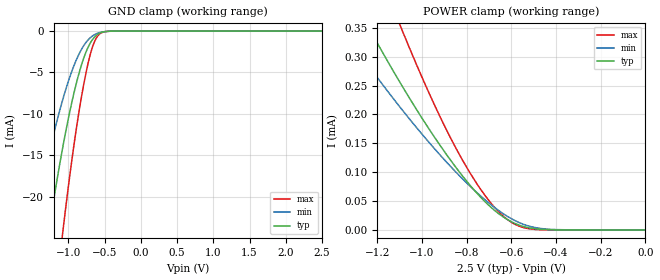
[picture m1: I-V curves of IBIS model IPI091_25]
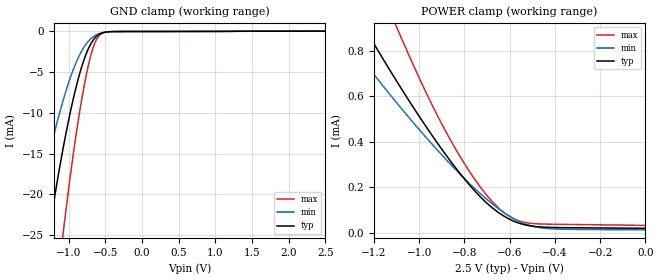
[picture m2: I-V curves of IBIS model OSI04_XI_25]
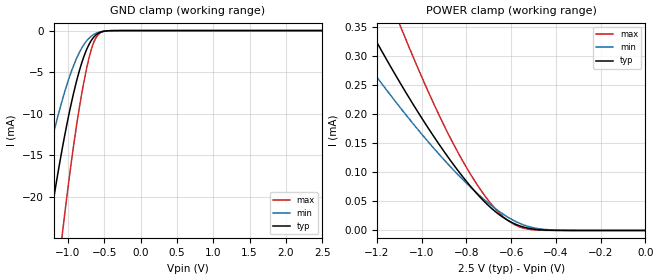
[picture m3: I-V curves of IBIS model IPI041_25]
| TEXAS INSTRUMENTS INCORPORATED
| Connectivity Solutions Group
| IBIS Model of TL16C752CRHB_2.5V
| 752C_RHB_2.5V
| This file contains package information for the following:
|  RHB 32-pin (QFN) package as [Component] 752CRHB_2.5V
| This device can be powered at the following Vccs:
|  2.5 Volt Vcc
| This file provides unique models under the [Model Selector] for each Vcc.
| For operation at a specific Vcc, select the appropriate model after each
| [Model Selector] keyword.
[IBIS Ver]   3.2
[Comment char]  |_char
[File Name]   752c_rhb_2_5v.ibs
[File Rev]   1 | a
[Date]   March 15, 2008
[Source]   Data created from TI-SPICE simulations at TI-CONN.
[Notes]   The following is an IBIS list for the 752C_RHB_2.5V.
   Please contact s-ly@ti.com with questions and
   comments concerning CONN IBIS models.
[Disclaimer] Property of Texas Instruments Incorporated.  Unauthorized
   reproduction and/or distribution is strictly prohibited.
   This product is protected under copyright law.
   Created  2003, (C) Copyright  2003, Texas Instruments
   Incorporated, All Rights Reserved
   UNLESS THERE IS A SIGNED, WRITTEN AGREEMENT TO THE
   CONTRARY, TEXAS INSTRUMENTS (TI) IS PROVIDING THE IBIS
   MODELS  AND WITHOUT ANY WARRANTY, EXPRESSED OR
   IMPLIED.  TI assumes no liability for:
   1) the accuracy of the IBIS models provided to your
   company;
   2) the proper functioning of these IBIS Models in your
   design or for any resulting applications; or
   3) infringement of patents, copyrights or intellectual
   property rights resulting from your use of these IBIS
   models.
   TI provides IBIS Models as a service to our customers.
   You and your company shall not distribute, sell or give
   these models to anyone else without prior written
   permission from TI.
   TI reserves the right to make changes to our products or
   to discontinue any semiconductor product or service
   without notice, and advises our customers to obtain the
   latest version of relevant information to verify, before
   placing orders, that the information being relied on is
   current.
   Please be aware that your receipt and use of the IBIS
   information provided shall serve as acceptance of these
   terms and conditions.  If you do not accept these terms,
   you should return or destroy the IBIS models and any
   other accompanying information immediately.
| Component 752C_2.5V_RHB 32-pin QFN
[Component]   752C_RHB_2.5V
[Manufacturer]   Texas Instruments, Inc.
[Package]
|   typ   min   max
R_pkg   0.03169   0.03002   0.03704
L_pkg   2.02289n   1.83543n   2.62435n
C_pkg   0.52087p   0.46196p   0.61212p
[Pin]   signal_name   model_name   R_pin   L_pin   C_pin
1   D6   IPI04_OPJ43   0.03132   1.96376n   0.50826p
2   D7   IPI04_OPJ43   0.03166   2.03022n   0.52764p
3   RXB   IPI041   0.03222   2.12197n   0.55702p
4   RXA   IPI041   0.03290   2.21862n   0.57989p
5   TXA   OPJ430   0.03010   1.83593n   0.46505p
6   TXB   OPJ430   0.03096   1.92107n   0.49718p
7   CSA   IPI041   0.03104   1.92183n   0.49798p
8   CSB   IPI041   0.03110   1.96691n   0.51031p
9   XTAL1   OSI04_XI   0.03077   1.83703n   0.47632p
10   XTAL2   OSI04   0.03175   1.92839n   0.50935p
11   IOW   IPI041   0.03007   1.83565n   0.46474p
12   GND   GND   0.03265   2.22076n   0.58208p
13   IOR   IPI041   0.03002   1.83657n   0.46196p
14   RTSB   OPJ430   0.03190   2.11324n   0.55339p
15   CTSB   IPI041   0.03704   2.62435n   0.54475p
16   A2   IPI041   0.03147   1.97163n   0.51867p
17   A1   IPI041   0.03142   1.92513n   0.50753p
18   A0   IPI041   0.03060   1.83543n   0.47574p
19   INTB   OPJ430   0.03159   2.04484n   0.53228p
20   INTA   OPJ430   0.03117   1.96768n   0.51149p
21   RTSA   OPJ430   0.03153   2.03432n   0.53110p
22   DTRA   OPJ430   0.03280   2.22331n   0.58366p
23   DTRB   OPJ430   0.03352   2.34940n   0.60960p
24   RESET   IPI091   0.03188   1.96764n   0.51741p
25   CTSA   IPI041   0.03373   2.35631n   0.61212p
26   VCC   POWER   0.03224   2.13122n   0.55769p
27   D0   IPI04_OPJ43   0.03191   2.05000n   0.53623p
28   D1   IPI04_OPJ43   0.03138   1.96454n   0.50911p
29   D2   IPI04_OPJ43   0.03132   1.92758n   0.49950p
30   D3   IPI04_OPJ43   0.03043   1.84011n   0.46416p
31   D4   IPI04_OPJ43   0.03039   1.83956n   0.46402p
32   D5   IPI04_OPJ43   0.03129   1.92740n   0.49881p
| Model IPI091
[Model Selector]   IPI091
IPI091_25   2.5 volt Vcc
| Model OSI04_XI
[Model Selector]   OSI04_XI
OSI04_XI_25   2.5 volt Vcc
| Model IPI041
[Model Selector]   IPI041
IPI041_25   2.5 volt Vcc
| Model IPI04_OPJ43
[Model Selector]   IPI04_OPJ43
IPI04_OPJ43_25   2.5 volt Vcc
| Model OPJ430
[Model Selector]   OPJ430
OPJ430_25   2.5 volt Vcc
| Model OSI04
[Model Selector]   OSI04
OSI04_25   2.5 volt Vcc
| Models and submodels in the file (6): IPI091_25 (Input), OSI04_XI_25 (Input), IPI041_25 (Input), IPI04_OPJ43_25 (I/O), OPJ430_25 (3-state), OSI04_25 (3-state)
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[Model]   IPI091_25
Model_type  Input
Vinl = 0
Vinh = 2.5
| variable   typ   min   max
C_comp   1.09pF   0.97pF   1.21pF
[Temperature Range]   40   125   -40
| Ambient temperature   25   110   -40
[Voltage range]   2.5   2.3   2.7
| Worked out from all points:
|   GND clamp passes 1 mA (typ) near -0.66 V on its own axis
|   POWER clamp passes 1 mA (typ) near -2.03 V on its own axis
[GND Clamp]
| IPI091_25
|   Voltage   I(typ)   I(min)   I(max)
-2.5V     -115mA     -79.72mA   -164.4mA
-1.485V   -37.43mA   -23.94mA   -59.12mA
-1.265V   -23.92mA   -14.77mA   -39.38mA
-1.08V    -14.2mA    -8.377mA   -24.56mA
-1.065V   -13.5mA    -7.923mA   -23.45mA
-955mV    -8.737mA   -4.937mA   -15.83mA
-830mV    -4.417mA   -2.392mA   -8.532mA
-730mV    -2.005mA   -1.091mA   -3.99mA
-635mV    -690.9uA   -415.3uA   -1.203mA
-560mV    -221.4uA   -161.8uA   -300.1uA
-440mV    -21.14uA   -26.42uA   -19.38uA
2.5V      179.9pA    7.156nA    49.54pA
[POWER Clamp]
| IPI091_25
|   Voltage   I(typ)   I(min)   I(max)
-2.5V     1.454mA    1.097mA    2.083mA
-1.36V    439.4uA    350.2uA    624.8uA
-1.235V   348.4uA    282.4uA    491.3uA
-1.095V   253.5uA    211.2uA    352uA
-1.075V   240.6uA    201.5uA    333.1uA
-945mV    161.4uA    141.3uA    217.5uA
-830mV    99.28uA    93.13uA    129uA
-720mV    49.87uA    53.05uA    61.07uA
-630mV    21.07uA    26.64uA    21.99uA
-550mV    6.466uA    10.43uA    4.583uA
-465mV    1.046uA    2.442uA    370.2nA
-31.11fV  179.9pA    1.684nA    54.24pA
[Model]   OSI04_XI_25
Model_type  Input
Vinl = 0
Vinh = 2.5
| variable   typ   min   max
C_comp   1.81pF   1.12pF   2.40pF
[Temperature Range]   40   125   -40
| Ambient temperature   25   110   -40
[Voltage range]   2.5   2.3   2.7
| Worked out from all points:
|   GND clamp passes 1 mA (typ) near -0.66 V on its own axis
|   POWER clamp passes 1 mA (typ) near -1.30 V on its own axis
[GND Clamp]
| OSI04_XI_25
|   Voltage   I(typ)   I(min)   I(max)
-2.5V     -117.2mA   -81mA      -167.9mA
-1.48V    -38.04mA   -24.27mA   -60.11mA
-1.26V    -24.32mA   -15mA      -40.01mA
-1.075V   -14.44mA   -8.535mA   -24.92mA
-1.06V    -13.72mA   -8.076mA   -23.8mA
-930mV    -8.097mA   -4.582mA   -14.76mA
-815mV    -4.206mA   -2.33mA    -8.111mA
-710mV    -1.776mA   -1.037mA   -3.434mA
-625mV    -669.3uA   -465.2uA   -1.116mA
-545mV    -205.3uA   -194.2uA   -270.4uA
-430mV    -40.49uA   -47uA      -53.13uA
2.5V      19.05uA    13.35uA    29.56uA
[POWER Clamp]
| OSI04_XI_25
|   Voltage   I(typ)   I(min)   I(max)
-2.5V     3.431mA    2.617mA    4.916mA
-1.355V   1.099mA    896.3uA    1.535mA
-1.24V    898.6uA    746.4uA    1.242mA
-1.22V    864.6uA    720.9uA    1.193mA
-1.095V   659.2uA    565.9uA    893.7uA
-935mV    416.4uA    380.2uA    546.2uA
-830mV    273.7uA    268.3uA    352.9uA
-720mV    148uA      163.2uA    188uA
-625mV    72.54uA    88.13uA    88.07uA
-555mV    40.52uA    47.83uA    50.59uA
-465mV    25.13uA    21.75uA    38.3uA
-31.11fV  19.05uA    12.27uA    31.94uA
[Model]   IPI041_25
Model_type  Input
Vinl = 0
Vinh = 2.5
| variable   typ   min   max
C_comp   1.10pF   0.98pF   1.21pF
[Temperature Range]   40   125   -40
| Ambient temperature   25   110   -40
[Voltage range]   2.5   2.3   2.7
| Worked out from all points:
|   GND clamp passes 1 mA (typ) near -0.66 V on its own axis
|   POWER clamp passes 1 mA (typ) near -2.03 V on its own axis
[GND Clamp]
| IPI041_25
|   Voltage   I(typ)   I(min)   I(max)
-2.5V     -115mA     -79.72mA   -164.4mA
-1.485V   -37.43mA   -23.94mA   -59.12mA
-1.265V   -23.92mA   -14.77mA   -39.38mA
-1.08V    -14.2mA    -8.377mA   -24.56mA
-1.065V   -13.5mA    -7.923mA   -23.45mA
-955mV    -8.737mA   -4.937mA   -15.83mA
-830mV    -4.417mA   -2.392mA   -8.532mA
-730mV    -2.005mA   -1.091mA   -3.99mA
-635mV    -690.9uA   -415.3uA   -1.203mA
-560mV    -221.4uA   -161.8uA   -300.1uA
-440mV    -21.14uA   -26.42uA   -19.38uA
2.5V      179.9pA    7.156nA    49.54pA
[POWER Clamp]
| IPI041_25
|   Voltage   I(typ)   I(min)   I(max)
-2.5V     1.454mA    1.097mA    2.083mA
-1.36V    439.4uA    350.2uA    624.8uA
-1.235V   348.4uA    282.4uA    491.3uA
-1.095V   253.5uA    211.2uA    352uA
-1.075V   240.6uA    201.5uA    333.1uA
-945mV    161.4uA    141.3uA    217.5uA
-830mV    99.28uA    93.13uA    129uA
-720mV    49.87uA    53.05uA    61.07uA
-630mV    21.07uA    26.64uA    21.99uA
-550mV    6.466uA    10.43uA    4.583uA
-465mV    1.046uA    2.442uA    370.2nA
-31.11fV  179.9pA    1.684nA    54.24pA
